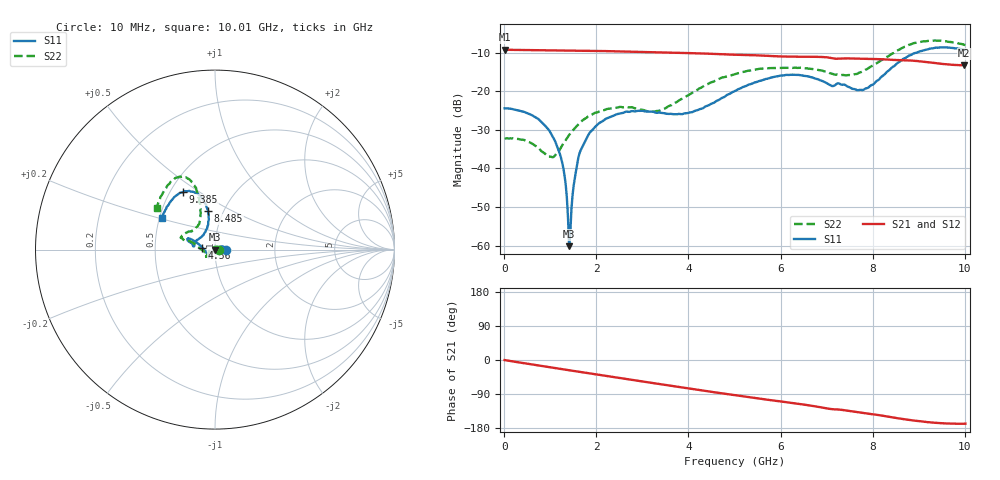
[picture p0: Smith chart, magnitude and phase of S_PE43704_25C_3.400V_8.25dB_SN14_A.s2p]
! Device ID: PE43704
! Dir: z:\PE43704\PE43704_Char_1_20130516\PE43704\AMB\3p400V\8p25dB
! Serial: 14
! Insertion: A
! Impedance: 50 ohm
! Temp: Amb
! VDD: 3.400V
! Attenuation Step: 8.25dB
! IDD: 1.140341e-01mA
#  Hz  S  RI  R  50
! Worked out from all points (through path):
!   401 points, 10 MHz to 10.01 GHz, reference 50 ohm
!   highest |S21| = -9.24 dB at 10 MHz (marker M1); lowest = -13.3 dB at 9.985 GHz (marker M2)
!   group delay of S21, straight-line fit = 48.5 ps
!   lowest |S11| = -60.1 dB at 1.41 GHz (marker M3), VSWR 1.00, Z = 50.1 - j0.0251 ohm
!   |S11| at or under -10 dB: start of sweep to 8.945 GHz
!   |S22| runs from -37.1 to -6.8 dB; largest |S21 - S12| = 0.0024
!   S11 on the Smith chart (normalised r, x): 10 MHz: 1.13, +0.00; 4.56 GHz: 0.87, +0.02; 8.485 GHz: 0.85, +0.38; 9.385 GHz: 0.58, +0.43; 10.01 GHz: 0.52, +0.20
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1e7  0.0602 0.000188  0.3451 -0.00122  0.3452 -0.00121  0.0244 0.000317
6.35e8  0.0447 0.017  0.3341 -0.073  0.334 -0.0728  0.0118 0.0167
1.035e9  0.0231 0.014  0.3201 -0.1158  0.32 -0.1156  -0.00752 0.0119
1.26e9  0.00993 0.00653  0.3091 -0.1391  0.3092 -0.139  -0.0196 0.00405
1.41e9  0.000952 -0.00025  0.3009 -0.1535  0.301 -0.1535  -0.0269 -0.00312
1.46e9  -0.00163 -0.00247  0.2982 -0.1583  0.298 -0.1581  -0.0289 -0.00569
1.56e9  -0.00708 -0.00607  0.2923 -0.1677  0.2923 -0.1676  -0.0329 -0.0108
1.685e9  -0.0131 -0.0129  0.2842 -0.1793  0.2842 -0.1792  -0.0375 -0.0171
1.885e9  -0.0211 -0.0218  0.2706 -0.1965  0.2706 -0.1963  -0.0417 -0.0264
2.235e9  -0.0288 -0.0342  0.2442 -0.224  0.2444 -0.2239  -0.0468 -0.036
3.36e9  -0.0375 -0.0375  0.1442 -0.286  0.1446 -0.2858  -0.0527 -0.0184
3.91e9  -0.0487 -0.0174  0.0905 -0.3006  0.0909 -0.3006  -0.083 0.00521
4.56e9  -0.0705 0.0116  0.026 -0.3038  0.0265 -0.3039  -0.1283 0.0422
5.01e9  -0.0952 0.0335  -0.0143 -0.2974  -0.014 -0.2976  -0.16 0.0487
5.96e9  -0.1453 0.062  -0.0908 -0.2685  -0.0897 -0.2689  -0.1892 0.0661
6.685e9  -0.1452 0.0436  -0.1442 -0.2398  -0.1444 -0.2393  -0.1758 0.0832
7.735e9  -0.0712 0.0762  -0.1987 -0.1751  -0.1987 -0.1754  -0.0859 0.1542
8.36e9  -0.0353 0.1853  -0.2223 -0.1284  -0.2214 -0.1296  -0.0872 0.2777
8.485e9  -0.0385 0.2142  -0.2264 -0.1176  -0.2248 -0.1184  -0.0947 0.3096
9.385e9  -0.1766 0.3218  -0.2239 -0.056  -0.2247 -0.0551  -0.2269 0.3922
9.985e9  -0.292 0.1836  -0.2129 -0.0446  -0.2142 -0.0444  -0.3204 0.239
1.001e10  -0.2969 0.1735  -0.2137 -0.0453  -0.2151 -0.0456  -0.3236 0.2314
